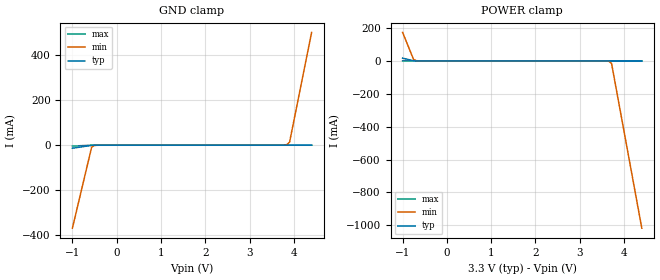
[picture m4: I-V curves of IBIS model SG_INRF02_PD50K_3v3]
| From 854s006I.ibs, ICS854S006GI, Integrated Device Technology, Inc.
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[Model] SG_INRF02_PD50K_3v3
Model_type   Input
Polarity   Non-Inverting
Vinl = 0.8V
Vinh = 2.0V
|   typ   min   max
C_comp   2pF   1.5pF   2.5pF
|   typ   min   max
[Voltage range]   3.3V   3.135V   3.465V
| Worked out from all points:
|   GND clamp passes 1 mA (typ) near -0.58 V on its own axis
|   POWER clamp passes 1 mA (typ) near -0.75 V on its own axis
[GND_clamp]
|Voltage   I (typ)   I (min)   I (max)
-999mV    -13.4mA    -368.6mA   -3.626mA
-564.6mV  -601.6uA   -8.535mA   -255.2uA
-502.5mV  -178.6uA   -1.359mA   -57.43uA
3.841V    80.46uA    2.38mA     71.23uA
3.904V    100uA      14.15mA    72.39uA
4.4V      714.2uA    501.6mA    81.74uA
[Power_clamp]
|Voltage   I (typ)   I (min)   I (max)
-999mV    16.9mA     173.7mA    1.118mA
-750.8mV  783.8uA    8.349mA    152.9uA
-688.7mV  242.8uA    1.5mA      91.39uA
3.531V    -4.598uA   -78.77uA   -1.227uA
3.655V    -9.731uA   -2.266mA   -3.529uA
3.717V    -26.95uA   -14.79mA   -4.681uA
4.4V      -924.5uA   -1.017A    -17.58uA
